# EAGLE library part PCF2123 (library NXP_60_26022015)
SPI Real time clock/calendar The PCF2123 is a CMOS1 Real-Time Clock (RTC) and calendar optimized for low power applications. Data is transferred serially via a Serial Peripheral Interface (SPI-bus) with a maximum data rate of 6.25 Mbit/s. An alarm and timer function is also available providing the possibility to generate a wake-up signal on an interrupt pin. An offset register allows fine tuning of the clock. AAL Eindhoven MK
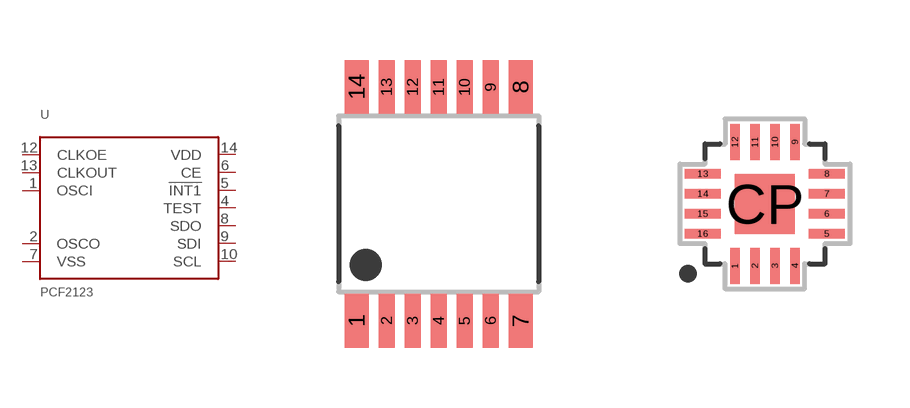
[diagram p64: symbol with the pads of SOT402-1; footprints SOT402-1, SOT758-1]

Designator prefix U

## PCF2123TS  [SOT402-1]
1  OSCI  pas
2  OSCO  pas
4  TEST  out
5  !INT1!  out
6  CE  in
7  VSS  pwr
8  SDO  out
9  SDI  in
10  SCL
12  CLKOE  in
13  CLKOUT  out
14  VDD  pwr

## PCF2123BS  [SOT758-1]
1  OSCO  pas
2  TEST  out
3  !INT1!  out
4  CE  in
5  VSS  pwr
8  SDO  out
9  SDI  in
10  SCL
11  CLKOE  in
12  CLKOUT  out
13  VDD  pwr
16  OSCI  pas

## Footprint SOT402-1 (pad centres in mm)
SOT402-1 TSSOP14: plastic thin shrink small outline package; 14 leads; body width 4.4 mm JEDEC: MO-153 IEC: ---
smd 0.6 x 1.35: 1 -2.05,-2.925; 7 2.05,-2.925; 8 2.05,2.925; 14 -2.05,2.925
smd 0.4 x 1.35: 2 -1.3,-2.925; 3 -0.65,-2.925; 4 0,-2.925; 5 0.65,-2.925; 6 1.3,-2.925; 9 1.3,2.925; 10 0.65,2.925; 11 0,2.925; 12 -0.65,2.925; 13 -1.3,2.925

## Footprint SOT758-1 (pad centres in mm)
SOT758-1 HVQFN16: plastic thermal enhanced very thin quad flat package; no leads; 16 terminals; body 3 x 3 x 0.85 mm JEDEC: MO-220 IEC: -- JEITA: --
smd 0.24 x 0.9: 1 -0.75,-1.55; 2 -0.25,-1.55; 3 0.25,-1.55; 4 0.75,-1.55; 9 0.75,1.55; 10 0.25,1.55; 11 -0.25,1.55; 12 -0.75,1.55
smd 0.9 x 0.24: 5 1.55,-0.75; 6 1.55,-0.25; 7 1.55,0.25; 8 1.55,0.75; 13 -1.55,0.75; 14 -1.55,0.25; 15 -1.55,-0.25; 16 -1.55,-0.75
smd 1.5 x 1.5: CP 0,0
